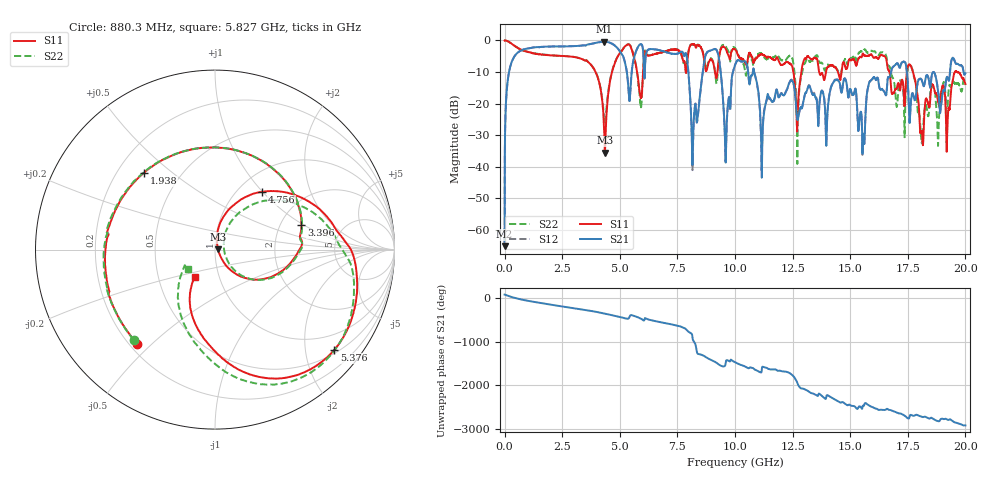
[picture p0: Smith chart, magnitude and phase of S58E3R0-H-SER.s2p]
!{S58E3R0}
!Johanson Technology Inc.
!www.johansontechnology.com
!Test Board Conditions:
!Substrate Type  RO4350B
!Substrate Thickness  60 mil
!Substrate Dk  3.66
!TL Type: GCPW
!TL Trace Width  115 mil
!TL Gap  52 mil
!Electrode orientation  Horizontal
!DUT TOPOLOGY	SERIES
!Mounting Pad LxW  55x428 mil
! Created Tue Apr 13 22:34:16 2021
# hz S ma R 50
! 2 Port Network Data from SP1.SP block
! freq  magS11  angS11  magS21  angS21  magS12  angS12  magS22  angS22
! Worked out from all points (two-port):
!   20001 points, 300 kHz to 20 GHz, reference 50 ohm
!   highest |S21| = -0.38 dB at 4.334 GHz (marker M1); lowest = -65.1 dB at 300 kHz (marker M2)
!   |S21| within 3 dB of the highest: 662.6 MHz to 5.002 GHz (4.34 GHz wide, 153 % of centre); 6.175 GHz to 6.869 GHz (693.6 MHz wide, 10.6 % of centre)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
!   lowest |S11| = -35.5 dB at 4.355 GHz (marker M3), VSWR 1.03, Z = 51.7 + j0.257 ohm
!   |S11| at or under -10 dB: 3.951 GHz to 4.662 GHz (711.1 MHz wide, 16.5 % of centre); 16.71 GHz to 17.46 GHz (751.9 MHz wide, 4.4 % of centre); 17.73 GHz to 19.54 GHz (1.815 GHz wide, 9.74 % of centre)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
!   |S22| runs from -39.1 to 0.0 dB; largest |S21 - S12| = 0.01
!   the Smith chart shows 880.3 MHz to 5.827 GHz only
!   S11 on the Smith chart (normalised r, x): 880.3 MHz: 0.23, -0.45; 1.938 GHz: 0.31, +0.40; 3.396 GHz: 2.61, +0.94; 4.756 GHz: 1.27, +0.99; 5.376 GHz: 0.58, -2.63; 5.827 GHz: 0.76, -0.24
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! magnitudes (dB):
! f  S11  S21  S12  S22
! 300 kHz  0.0  -65.1  -64.9  0.0
! 183.3 MHz  -0.4  -10.4  -10.3  -0.4
! 880.3 MHz  -3.4  -2.7  -2.7  -3.4
! 1.938 GHz  -4.7  -1.9  -1.9  -4.6
! 3.334 GHz  -5.8  -1.6  -1.6  -5.8
! 3.396 GHz  -6.0  -1.6  -1.6  -6.0
! 4.334 GHz  -31.4  -0.4  -0.4  -25.4
! 4.355 GHz  -35.5  -0.4  -0.4  -26.1
! 4.756 GHz  -7.7  -1.5  -1.5  -7.6
! 5.376 GHz  -1.2  -15.4  -15.4  -1.2
! 5.827 GHz  -14.5  -1.6  -1.6  -14.6
! 6.667 GHz  -4.0  -3.0  -3.0  -4.0
! 7.84 GHz  -8.5  -4.1  -4.1  -8.4
! 8.17 GHz  -1.2  -34.8  -35.3  -1.3
! 8.796 GHz  -8.7  -3.7  -3.7  -8.0
! 9.592 GHz  -2.6  -38.6  -38.2  -1.8
! 10 GHz  -2.8  -7.9  -7.9  -2.5
! 11.18 GHz  -4.4  -34.2  -31.0  -4.5
! 13.33 GHz  -6.0  -16.7  -16.5  -6.2
! 16.67 GHz  -9.5  -11.6  -11.6  -8.1
! 18.11 GHz  -29.1  -12.6  -12.6  -32.4
! 20 GHz  -13.8  -10.4  -10.3  -14.1
